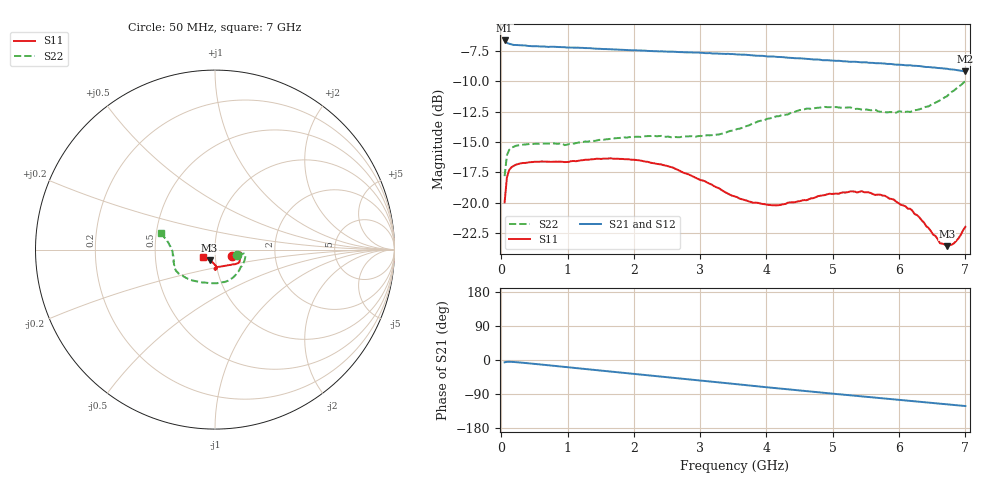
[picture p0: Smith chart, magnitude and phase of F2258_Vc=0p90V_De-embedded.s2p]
! Integrated Device Technology
! Corporate Headquarters
! 6024 Silver Creek Valley Road
! San Jose, CA 95138  USA
! Phone:  1-408-284-8200
! Toll Free:  1-800-223-1366
! Webpage:  http://www.idt.com/
! Timing and RF Division
! 515 Groton Road, Suite 102
! Westford, MA 01886-6024
! Device:  F2258
! Description: Voltage Variable RF Attenuator
! Frequency:  50.0 -  6000.00 MHz
! Package:  3x3 mm Thin QFN Plastic Package: 16 pin
! Ports:  2 RF, 2 DC
!  Pin  1  = NC
!  Pin  2  = NC
!  Pin  3  = RF2  = Port 2
!  Pin  4  = GND
!  Pin  5  = Vdd
!  Pin  6  = NC
!  Pin  7  = VCTRL
!  Pin  8  = NC
!  Pin  9  = GND
!  Pin 10  = RF1  = Port 1
!  Pin 11  = NC
!  Pin 12  = NC
!  Pin 13  = NC
!  Pin 14  = NC
!  Pin 15  = NC
!  Pin 16  = NC
! Vcntrl:  0.900 Volts
! Vdd:  +3.300 Volts
! Current:  1.148 mA
! Data:  The device was measured on a the F2258 evaluation board which has
!  individual transmission lines to the RF pins.  Data was collected
!  using a calibrated network analyzer.  The evaluation board was
!  de-embedded using a TRL calibration technique.
!  The reference plane is the edge of the package pin.
! Misc:  SN 10
!  Action Tracker AT0285
! Date Measured:  2014-12-10
! Date:  2016-01-13  MJV
! Note:
!  Integrated Device Technology supplies this data as a sample of measured
!  data at the package pin for this product.  Your particular data for this
!  product may vary.
!  Data was taken at 25 degrees C.
!  Integrated Device Technology reserves the right to change this data at anytime.
!Freq_(GHz)  S11M_(dB)  S11P_(deg)  S21M_(dB)  S21P_(deg)  S12M_(dB)  S12P_(deg)  S22M_(dB)  S22P_(deg)
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# GHz S dB R 50
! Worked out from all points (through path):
!   201 points, 50 MHz to 7 GHz, reference 50 ohm
!   highest |S21| = -6.67 dB at 50 MHz (marker M1); lowest = -9.2 dB at 7 GHz (marker M2)
!   group delay of S21, straight-line fit = 47.8 ps
!   lowest |S11| = -23.5 dB at 6.722 GHz (marker M3), VSWR 1.14, Z = 46.8 - j5.56 ohm
!   |S11| at or under -10 dB: start of sweep to end of sweep
!   |S22| runs from -17.8 to -10.0 dB; largest |S21 - S12| = 0.0023
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0.05  -19.95 -20.3  -6.67 -6.0  -6.69 -6.1  -17.80 -14.2
0.08475  -17.90 -10.0  -6.87 -4.8  -6.89 -4.8  -16.09 -8.3
0.1195  -17.29 -7.2  -6.94 -4.6  -6.96 -4.7  -15.64 -7.8
0.189  -16.95 -6.4  -7.04 -5.2  -7.02 -5.2  -15.38 -8.8
0.43225  -16.66 -9.0  -7.13 -9.0  -7.12 -9.0  -15.16 -15.6
0.9535  -16.65 -18.8  -7.22 -18.3  -7.21 -18.3  -15.26 -33.3
1.2315  -16.49 -22.3  -7.28 -23.2  -7.27 -23.2  -15.00 -41.9
1.6485  -16.34 -26.7  -7.39 -30.4  -7.38 -30.4  -14.74 -53.7
2.37825  -16.82 -32.7  -7.57 -43.0  -7.54 -43.0  -14.51 -73.6
3.0385  -18.16 -43.1  -7.69 -54.7  -7.67 -54.7  -14.52 -95.9
3.525  -19.46 -57.5  -7.80 -63.4  -7.79 -63.4  -14.01 -115.3
3.803  -19.99 -68.8  -7.89 -68.4  -7.87 -68.4  -13.46 -125.8
4.1505  -20.20 -80.2  -8.01 -74.5  -8.01 -74.5  -12.89 -136.3
4.7065  -19.61 -90.3  -8.23 -84.0  -8.22 -84.0  -12.26 -149.1
5.43625  -19.03 -88.0  -8.46 -96.0  -8.46 -96.0  -12.34 -160.9
5.85325  -19.65 -85.0  -8.59 -102.8  -8.59 -102.8  -12.54 -169.5
6.166  -20.48 -86.3  -8.70 -108.0  -8.72 -107.9  -12.53 -176.8
6.3745  -21.60 -91.6  -8.82 -111.5  -8.81 -111.5  -12.16 177.9
6.61775  -23.31 -106.0  -8.94 -115.4  -8.93 -115.4  -11.59 171.3
6.722  -23.55 -117.0  -8.99 -117.2  -8.99 -117.2  -11.25 168.5
6.82625  -23.32 -129.5  -9.06 -118.8  -9.07 -118.8  -10.79 166.6
7  -21.96 -150.4  -9.19 -121.5  -9.18 -121.6  -9.98 163.1
